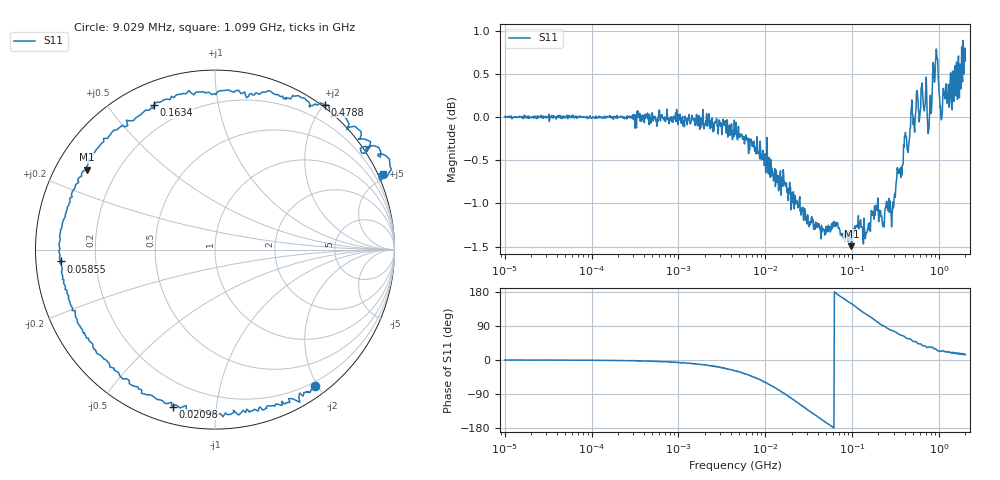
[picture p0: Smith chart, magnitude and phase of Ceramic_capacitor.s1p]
#  HZ  Z  MA  R  50.0
! 1 port S parameter measurement of a 10 nF X7R ceramic capacitor mounted in a 0805 case
! Kemet C0805C103K5RACAUTO
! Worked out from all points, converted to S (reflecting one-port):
!   1000 points, 10 kHz to 2 GHz, reference 50 ohm
!   lowest |S11| = -1.5 dB at 97.81 MHz (marker M1), VSWR 11.65, Z = 4.64 + j14.2 ohm
!   phase of S11 starts at -0 deg and turns -346 deg over the sweep
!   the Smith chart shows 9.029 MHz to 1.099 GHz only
!   S11 on the Smith chart (normalised r, x): 9.029 MHz: 0.14, -1.97; 20.98 MHz: 0.08, -0.76; 58.55 MHz: 0.07, -0.04; 163.4 MHz: 0.10, +0.66; 478.8 MHz: -0.03, +2.01; 1.099 GHz: -0.32, +4.62
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10000  684 -97.9
46056.62  264.7 -75.0
212121.2  82.95 -91.0
976958.5  18.21 -88.8
2135412  8.163 -89.1
4499541  3.93 -89.0
6412862  2.744 -85.7
9028786  1.973 -86.0
1.526869e7  1.123 -84.7
2.072336e7  0.7777 -83.3
2.097812e7  0.7675 -84.1
2.582107e7  0.5898 -81.5
3.547636e7  0.3555 -77.2
5.854621e7  0.08364 -27.1
7.032243e7  0.1113 48.3
9.544479e7  0.2801 72.7
9.780587e7  0.2981 71.9
1.233631e8  0.454 79.4
1.633921e8  0.6659 81.6
2.505837e8  1.107 83.1
4.395864e8  1.862 86.8
4.78838e8  2.01 90.9
6.039612e8  2.564 90.5
7.902208e8  3.299 93.0
9.150071e8  3.824 99.5
1.008963e9  4.949 93.8
1.099055e9  4.634 93.9
2e9  7.931 107.5
